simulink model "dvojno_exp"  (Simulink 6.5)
settings: Solver=FixedStepDiscrete  StartTime=0.0  StopTime=50e-6  RelTol=1e-6
undefined symbols (not defined in the file or in its folder): blocks, Discrete, powergui, ZData
libraries: powerlib x6

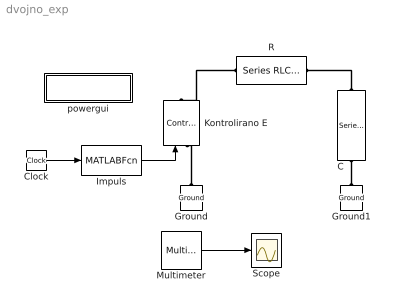
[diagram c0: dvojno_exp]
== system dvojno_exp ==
  C : powerlib/Elements/Series RLC Branch  Orientation=down  DialogController=PMDialogs.PMDefaultMaskDlg  PhysicalDomain=powersysdomain  SubClassName=unknown  LeftPortType=p1  RightPortType=p1  LConnTagsString=__new0  RConnTagsString=__new0  BranchType=C  Resistance=1  Inductance=1e-3  SetiL0=off  InitialCurrent=0  Capacitance=10e-9  Setx0=on  InitialVoltage=0  Measurements=Branch voltage
  Clock : Clock
  Ground : powerlib/Elements/Ground  Orientation=down  DialogController=PMDialogs.PMDefaultMaskDlg  PhysicalDomain=powersysdomain  SubClassName=unknown  LeftPortType=p1  RightPortType=p1  LConnTagsString=a
  Ground1 : powerlib/Elements/Ground  Orientation=down  DialogController=PMDialogs.PMDefaultMaskDlg  PhysicalDomain=powersysdomain  SubClassName=unknown  LeftPortType=p1  RightPortType=p1  LConnTagsString=a
  Impuls : MATLABFcn  MATLABFcn=100e3 * (exp(-1.38e4*u) - exp(-2.7e6*u))  OutputSignalType=real
  Kontrolirano E : powerlib/Electrical Sources/Controlled Voltage Source  Orientation=up  DialogController=PMDialogs.PMDefaultMaskDlg  SystemSampleTime=-1  Initialize=on  Source_Type=AC  Amplitude=0  Phase=0  Frequency=0  Measurements=Voltage
  Multimeter : powerlib/Measurements/Multimeter  SystemSampleTime=-1  PhasorSimulation=off  OutputType=Complex  sel=[2 1]  L=2  Gain=[1 1]  yselected={'Usrc: Kontrolirano E','Ub: C'};  PSBOutputType=1  PSBequivalent=0  AxesSetting=[0,0.1,-100,100]  Display=0  SavedBlockNames=-11
  R : powerlib/Elements/Series RLC Branch  DialogController=PMDialogs.PMDefaultMaskDlg  PhysicalDomain=powersysdomain  SubClassName=unknown  LeftPortType=p1  RightPortType=p1  LConnTagsString=__new0  RConnTagsString=__new0  BranchType=R  Resistance=100  Inductance=1e-3  SetiL0=on  InitialCurrent=0  Capacitance=1e-6  Setx0=off  InitialVoltage=0  Measurements=None
  Scope : Scope
  powergui : Subsystem  AncestorBlock=powerlib/powergui  InitFcn=powergui( 'InitFcn_Callback' , gcb , 0 , [ ] );  mask(PSB option menu block){SimulationMode=Discrete, SampleTime=0.05e-6, echomessages=off, RestoreLinks=warning, x0status=blocks, Frange=[0:2:500], Ylog=off, Xlog=on, ShowGrid=off, save=off, variable=ZData, structure=, ZoomFFT=on, StartTime=0.0, cycles=1, DisplayStyle=1, fundamental=60, FreqAxis=off, MaxFrequency=1000, frequencyindice=0, frequencyindicesteady=1, RmsSteady=1, display=off, Ts=0, frequency=60, methode=off, HookPort=off, Interpol=off}
      mask prompts: SimulationMode "Simulation mode"; SampleTime "Sample time Ts (when simulation mode is Discrete) (s)"; echomessages "Echo  Messages"; RestoreLinks "Restore disabled links"; x0status "Initial electrical states status"; Frange "Impedance tool: Frequency Range"; Ylog "Impedance tool: Log impedance"; Xlog "Impedance tool: log Frequency"; ShowGrid "Impedance tool: grid"; save "Impedance tool: Save Data To Workspace"; variable "Impedance tool: Variable Name"; structure "Structure Name (PSBFFTSCOPE)"; ZoomFFT "ZoomFFT (PSBFFTSCOPE)"; StartTime "Start Time (PSBFFTSCOPE)"; cycles "Cycles (PSBFFTSCOPE)"; DisplayStyle "Display style (PSBFFTSCOPE)"; fundamental "Fundamental (PSBFFTSCOPE)"; FreqAxis "Frequency Axis (PSBFFTSCOPE)"; MaxFrequency "Max Frequency (PSBFFTSCOPE)"; frequencyindice "Load flow frequency (Hz)"; frequencyindicesteady "Frequency indice (STEADYSTATE)"; RmsSteady "RMS display (STEADYSTATE)"; display "Display Results"; Ts "OBSOLETE 1"; frequency "Phasor frequency (Hz)"; methode "Phasor simulation"; HookPort "Hook port"; Interpol "Interpolate"
      mask init:
      | powerlibroot = which('powersysdomain');
      | PSBroot = powerlibroot(1:end-16);
      | %
      | switch SimulationMode
      | 	case 1
      | 		message=sprintf('Continuous');
      | 	case 2
      |         SampleTimeeval=evalin('base',SampleTime,'NaN');
      |         if isnan(SampleTimeeval)
      |             message=sprintf('Warning !!,\nUndefined sample time');
      |         else
      |             message=sprintf('Discrete,\nTs = %.4g s.',SampleTimeeval);
      |         end
      | 	case 3
      | 		message=sprintf('Phasors');
      | end
      | if strcmp(bdroot,'powerlib')
      |   message='powergui';
      | end
      | power_initmask();
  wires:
  Impuls/1 -> Kontrolirano E/1
  Clock/1 -> Impuls/1
  Multimeter/1 -> Scope/1
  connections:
  Ground/LConn1 -- Kontrolirano E/LConn1
  R/LConn1 -- Kontrolirano E/RConn1
  C/LConn1 -- R/RConn1
  Ground1/LConn1 -- C/RConn1

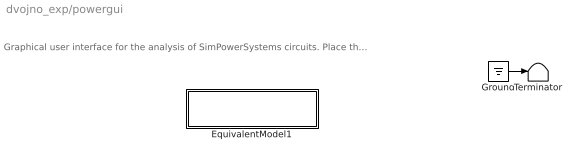
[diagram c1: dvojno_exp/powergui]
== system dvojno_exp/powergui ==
  note: Graphical user interface for the analysis of SimPowerSystems circuits. Place the Powergui block in the top-level of your model and double-click on it to open the GUI.
  EquivalentModel1 : Subsystem
  Ground : Ground
  Terminator : Terminator
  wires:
  Ground/1 -> Terminator/1

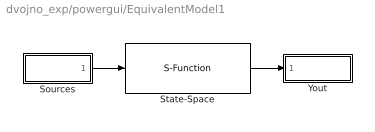
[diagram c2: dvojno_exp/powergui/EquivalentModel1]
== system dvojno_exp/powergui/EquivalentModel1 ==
  Sources : Subsystem
  State-Space : S-Function  FunctionName=sfun_spssw_discc  Parameters=Ts,A, B, C, D, x0
  Yout : Subsystem
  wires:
  Sources/1(u) -> State-Space/1
  State-Space/1 -> Yout/1(v,i)

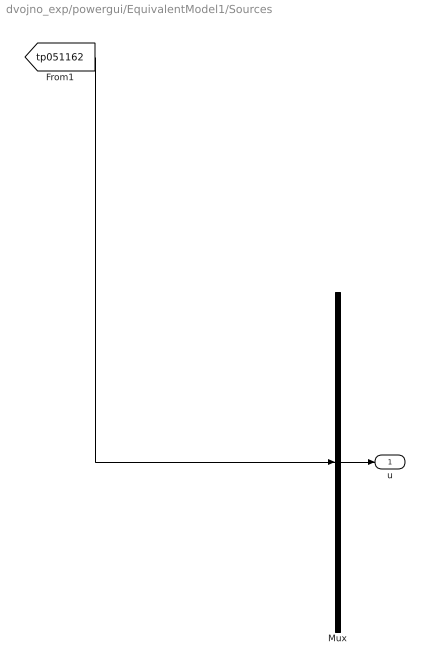
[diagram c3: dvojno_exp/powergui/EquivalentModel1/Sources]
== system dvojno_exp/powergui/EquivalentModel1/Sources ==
  Mux : Mux  Inputs=1
  u : Outport
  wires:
  Mux/1 -> u/1
  [tp051162] -> Mux/1

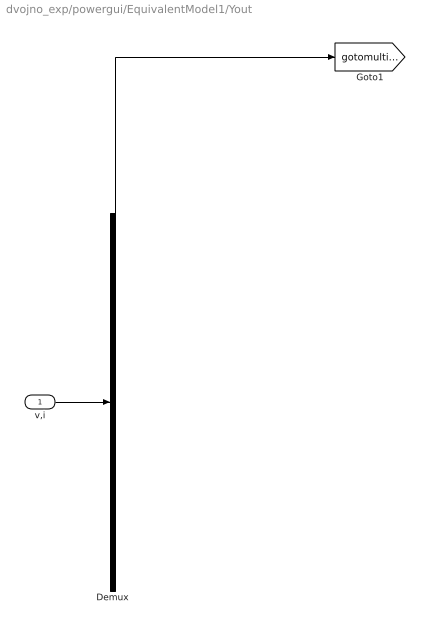
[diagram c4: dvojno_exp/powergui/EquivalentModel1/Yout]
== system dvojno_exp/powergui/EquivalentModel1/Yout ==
  v,i : Inport
  Demux : Demux  Outputs=1
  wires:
  v,i/1 -> Demux/1
  Demux/1 -> [gotomultimeterPSB]
